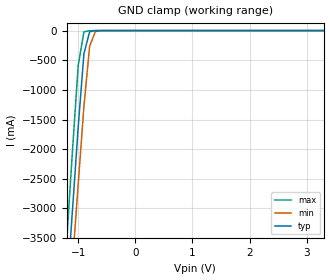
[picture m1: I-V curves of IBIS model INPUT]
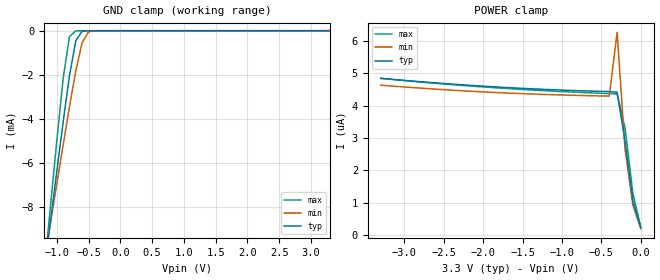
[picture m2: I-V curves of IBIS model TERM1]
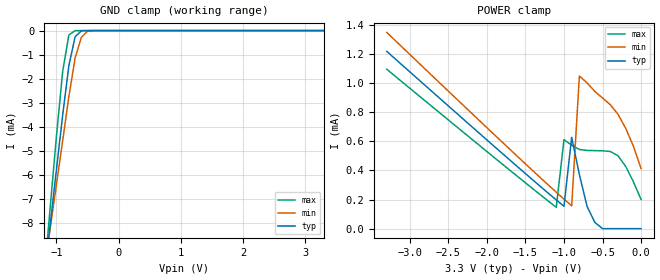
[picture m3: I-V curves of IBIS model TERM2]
|   PERICOM SEMICONDUCTOR CORP
|   IBIS Model of PI3USB102E
|   Product Family: PI3USB
|   TDFN (ZL) Package
[IBIS Ver] 3.2
[Comment char] |_char
[File Name] pi3usb102_zl_33v.ibs
[File Rev] 1.0
[Source] File originated at Pericom Semiconductor Corp.
[Date] 02/03/21
[Disclaimer] (C) Copyright PERICOM Semiconductor Corporation
   All rights reserved
  Pericom Semiconductor Corporation hereby grants the user of
  this IBIS model a non-exclusive, nontransferable license to
  use this IBIS model under the following terms.
  This IBIS model is provided on an "AS IS" basis and Pericom
  makes absolutely no warranty with respect to the information
  contained herein. PERICOM DISCLAIMS AND CUSTOMER WAIVES ALL
  WARRANTIES, EXPRESSED OR IMPLIED, INCLUDING WARRANTIES OF
  MERCHANTABILITY OR FITNESS FOR A PARTICULAR PURPOSE. The
  entire risk as to quality and performance is with the customer.
  Accordingly, in no event shall the company be liable for any
  damages, whether in contract or tort, including any lost
  profits or other incidental, consequential, exemplary, or
  punitive damages arising out of the use or application of the
  IBIS model provided in this package. Further, Pericom reserves
  the right to make changes without notice to any product herein
  to improve reliability, function, or design. Pericom does not
  convey any license under patent rights or any other intellectual
  property rights, including those of third parties.
  The user is granted this license only to use the IBIS model
  and is not granted rights to sell, load, rent, lease or license
  the IBIS model in whole or in part, or in modified form to anyone
  other than user. User may modify the IBIS model to suit its specific
  application but rights to derivative works and such modifications
  shall belong to Pericom.
  Pericom is not obligated to provide maintenance or support
  for the licensed IBIS model.
  Contact Pericom at ATTN: APPLICATION ENGINEERING / IBIS MODELS
  1545 Barber Lane Milpitas, CA 95035 USA.
[Component] PI3USB102E
[Manufacturer] Pericom Semiconductor Corp.
[Package]
| variable   typ   min   max
R_pkg   0.02854ohm   NA   NA
L_pkg   0.40283nH   NA   NA
C_pkg   0.04881pF   NA   NA
[Pin]   signal_name   model_name   R_pin   L_pin   C_pin
1   Y+   TERM1   0.027628   0.38515nH   0.058255pF
2   Y-   TERM1   0.027704   0.38506nH   0.057097pF
3   GND   GND   0.028167   0.43415nH   0.038030pF
4   M-   TERM2   0.027796   0.43415nH   0.041442pF
5   M+   TERM2   0.028245   0.42982nH   0.038022pF
6   D-   TERM2   0.027468   0.38133nH   0.056889pF
7   D+   TERM2   0.027577   0.38090nH   0.057154pF
8   OE#   INPUT   0.028352   0.44496nH   0.038136pF
9   VDD   POWER   0.028596   0.40988nH   0.041595pF
10   SEL   INPUT   0.028574   0.43936nH   0.038064pF
[Series Switch Groups]
On 1 /
[Series Pin Mapping]   pin_2   model_name  function_table_group
1   5   SWITCH1   1
1   7   SWITCH1   1
2   4   SWITCH1   1
2   6   SWITCH1   1
|   Model SWITCH1
[Model] SWITCH1
Model_type Series_switch
| variable   typ   min   max
C_comp   5.5pF   5.0pF   6.0pF
[Voltage Range]   3.30V   3.00V   3.60V
[GND Clamp Reference]   0.00V   0.00V   0.00V
[POWER Clamp Reference]   3.30V   3.00V   3.60V
[On]
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[OFF]
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| Models and submodels in the file (4): INPUT (Input), SWITCH1 (Series_switch), TERM1 (Terminator), TERM2 (Terminator)
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|   Model INPUT
[Model] INPUT
Model_type Input
Vinl = 0.80V
Vinh = 1.60V
| variable   typ   min   max
C_comp   2.2pF   2.0pF   2.4pF
[Voltage Range]   3.30V   3.00V   3.60V
[GND Clamp Reference]   0.00V   0.00V   0.00V
[POWER Clamp Reference]   3.30V   3.00V   3.60V
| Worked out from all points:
|   GND clamp passes 1 mA (typ) near -0.69 V on its own axis
[GND Clamp]
| Voltage   I(typ)   I(min)   I(max)
-3.3V     -33.77A    -32.86A    -34.97A
-1.2V     -4.421A    -5.225A    -3.521A
-1.1V     -3.024A    -3.909A    -2.024A
-1V       -1.627A    -2.593A    -590.2mA
-900mV    -392.9mA   -1.281A    -21.51mA
-800mV    -19.31mA   -264.3mA   -1.687mA
-700mV    -1.083mA   -16.92mA   -221.4uA
-500mV    -7.122uA   -64.68uA   -357.2nA
3.3V      79.58pA    126.9pA    79.21pA
[POWER Clamp]   |Note: Vtable = Vcc - Voutput
| Voltage   I(typ)   I(min)   I(max)
-3.3V     0A         0A         0A
0V        0A         0A         0A
|   Model TERM1
[Model] TERM1
Model_type Terminator
| variable   typ   min   max
C_comp   2.4pF   2.2pF   2.6pF
[Voltage Range]   3.30V   3.00V   3.60V
[GND Clamp Reference]   0.00V   0.00V   0.00V
[POWER Clamp Reference]   3.30V   3.00V   3.60V
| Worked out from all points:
|   GND clamp passes 1 mA (typ) near -0.73 V on its own axis
[GND Clamp]
| Voltage   I(typ)   I(min)   I(max)
-3.3V     -2.112A    -2.277A    -1.944A
-1.2V     -10.97mA   -10.56mA   -11.01mA
-1.1V     -8.698mA   -8.771mA   -8.02mA
-1V       -6.421mA   -6.985mA   -5.031mA
-900mV    -4.171mA   -5.207mA   -2.198mA
-800mV    -2.046mA   -3.462mA   -268.5uA
-700mV    -450uA     -1.82mA    -6.61uA
-600mV    -22.75uA   -542.3uA   -754.6nA
-500mV    -1.041uA   -52.26uA   -39.76nA
-400mV    -50.2nA    -2.787uA   -3.122nA
3.3V      223.8nA    6.259uA    9.091nA
[POWER Clamp]   |Note: Vtable = Vcc - Voutput
| Voltage   I(typ)   I(min)   I(max)
-3.3V     4.838uA    4.629uA    4.841uA
-1.8V     4.57uA     4.398uA    4.542uA
-400mV    4.43uA     4.292uA    4.369uA
-300mV    4.412uA    6.259uA    4.356uA
-200mV    2.914uA    2.663uA    3.316uA
-100mV    1.065uA    918.1nA    1.29uA
0V        223.8nA    197.2nA    252.8nA
|   Model TERM2
[Model] TERM2
Model_type Terminator
| variable   typ   min   max
C_comp   2.4pF   2.2pF   2.6pF
[Voltage Range]   3.30V   3.00V   3.60V
[GND Clamp Reference]   0.00V   0.00V   0.00V
[POWER Clamp Reference]   3.30V   3.00V   3.60V
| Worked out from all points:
|   GND clamp passes 1 mA (typ) near -0.76 V on its own axis
|   POWER clamp passes 1 mA (typ) near -2.84 V on its own axis
[GND Clamp]
| Voltage   I(typ)   I(min)   I(max)
-3.3V     -1.254A    -1.324A    -1.182A
-1.2V     -10.3mA    -9.968mA   -10.28mA
-1.1V     -8.04mA    -8.18mA    -7.32mA
-1V       -5.765mA   -6.381mA   -4.381mA
-900mV    -3.507mA   -4.566mA   -1.697mA
-800mV    -1.449mA   -2.735mA   -179.2uA
-700mV    -256.4uA   -1.138mA   -5.114uA
-600mV    -12.66uA   -286.8uA   -248.5nA
-500mV    -484.8nA   -25.65uA   -6.57nA
3.3V      5.177nA    21.87nA    5.124nA
[POWER Clamp]   |Note: Vtable = Vcc - Voutput
| Voltage   I(typ)   I(min)   I(max)
-3.3V     1.218mA    1.348mA    1.095mA
-1.1V     197.4uA    250.3uA    146.8uA
-1V       153.7uA    203.1uA    611uA
-900mV    627.6uA    156.9uA    573uA
-800mV    370.7uA    1.048mA    543.9uA
-700mV    152.7uA    1.001mA    537.2uA
-600mV    43.32uA    942.8uA    536.1uA
-500mV    161.2nA    897.4uA    534.7uA
-300mV    6.441nA    786.4uA    501.4uA
-200mV    5.561nA    690.3uA    428.1uA
-100mV    5.353nA    567.8uA    323.5uA
0V        5.177nA    413.4uA    201.2uA
